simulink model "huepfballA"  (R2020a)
settings: Solver=ode45  StartTime=0.0  StopTime=20  RelTol=1e-3  EnableMultiTasking=on

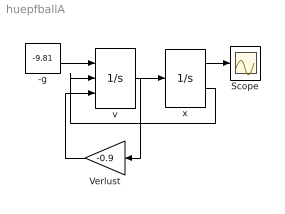
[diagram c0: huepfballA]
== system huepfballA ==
  note: .
  -g : Constant  Value=-9.81
  Scope : Scope
  Verlust : Gain  Gain=-0.9  SaturateOnIntegerOverflow=on
  v : Integrator  ExternalReset=falling  InitialConditionSource=external  LowerSaturationLimit=0
  x : Integrator  InitialCondition=20  LimitOutput=on  UpperSaturationLimit=Inf  LowerSaturationLimit=0  ShowSaturationPort=on
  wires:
  v/1 -> x/1, Verlust/1
  x/1 -> Scope/1
  -g/1 -> v/1
  x/2 -> v/2
  Verlust/1 -> v/3
